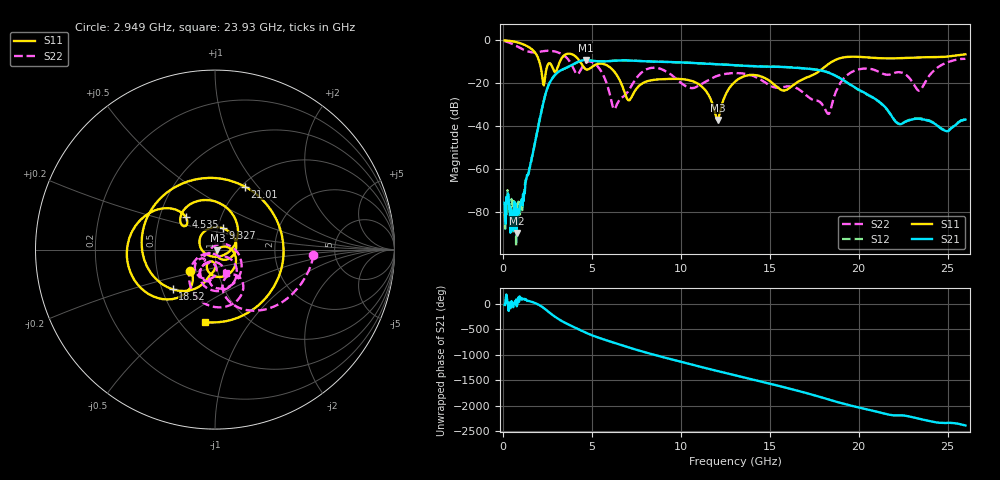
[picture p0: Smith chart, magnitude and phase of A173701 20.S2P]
!  2-Port S-parameters saved by WinCal
! VAR MeasName=S-Parameters (CALIBRATED_DATA) read from VNA (N5245A)
! VAR MeasDate=2017-6-7 10:29:41
! VAR NAME=A173701 20
! VAR FILENAME=A173701 20.S2P
! VAR DATE=2017-6-7 10:29:41
! VAR PHYS_PORTS=1,2
# Hz S DB R 50
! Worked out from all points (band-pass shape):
!   801 points, 100 MHz to 26 GHz, reference 50 ohm
!   highest |S21| = -9.17 dB at 4.665 GHz (marker M1); lowest = -89.7 dB at 779.9 MHz (marker M2)
!   |S21| within 3 dB of the highest: 3.719 GHz to 14.5 GHz (10.78 GHz wide, 118 % of centre); 14.51 GHz to 14.75 GHz (235 MHz wide, 1.61 % of centre)
!   lowest |S11| = -37.0 dB at 12.08 GHz (marker M3), VSWR 1.03, Z = 51.4 - j0.451 ohm
!   |S11| at or under -10 dB: 2.058 GHz to 3.198 GHz (1.141 GHz wide, 43.4 % of centre); 4.348 GHz to 18.48 GHz (14.13 GHz wide, 124 % of centre)
!   |S22| runs from -34.2 to -0.3 dB; largest |S21 - S12| = 0.0039
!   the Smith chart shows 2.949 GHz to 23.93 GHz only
!   S11 on the Smith chart (normalised r, x): 2.949 GHz: 0.74, -0.18; 4.535 GHz: 0.68, +0.26; 9.327 GHz: 1.06, +0.26; 18.52 GHz: 0.57, -0.28; 21.01 GHz: 1.04, +0.86; 23.93 GHz: 0.65, -0.63
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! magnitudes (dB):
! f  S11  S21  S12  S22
! 100 MHz  0.0  -75.6  -80.4  -0.3
! 779.9 MHz  -0.8  -89.7  -76.2  -2.7
! 1.039 GHz  -1.5  -76.6  -74.5  -3.8
! 2.269 GHz  -20.2  -29.3  -29.3  -5.0
! 2.949 GHz  -14.8  -15.9  -15.9  -5.2
! 4.438 GHz  -11.1  -9.4  -9.4  -12.8
! 4.535 GHz  -12.3  -9.2  -9.3  -11.5
! 4.665 GHz  -13.4  -9.2  -9.2  -10.4
! 6.284 GHz  -14.7  -9.4  -9.5  -32.0
! 7.093 GHz  -27.9  -9.4  -9.3  -23.1
! 8.744 GHz  -18.2  -9.9  -9.9  -13.0
! 9.327 GHz  -18.0  -10.0  -10.1  -15.2
! 11.11 GHz  -21.0  -10.6  -10.7  -20.6
! 12.08 GHz  -37.0  -11.1  -11.1  -16.5
! 13.05 GHz  -19.2  -11.6  -11.6  -15.2
! 17.39 GHz  -16.3  -13.4  -13.3  -27.6
! 18.52 GHz  -9.8  -15.7  -15.7  -29.1
! 19.43 GHz  -7.6  -20.1  -20.1  -15.7
! 21.01 GHz  -8.2  -27.7  -27.8  -14.2
! 21.69 GHz  -8.4  -33.2  -33.3  -15.9
! 23.93 GHz  -7.8  -37.4  -37.3  -16.9
! 26 GHz  -6.5  -36.9  -36.9  -8.6
